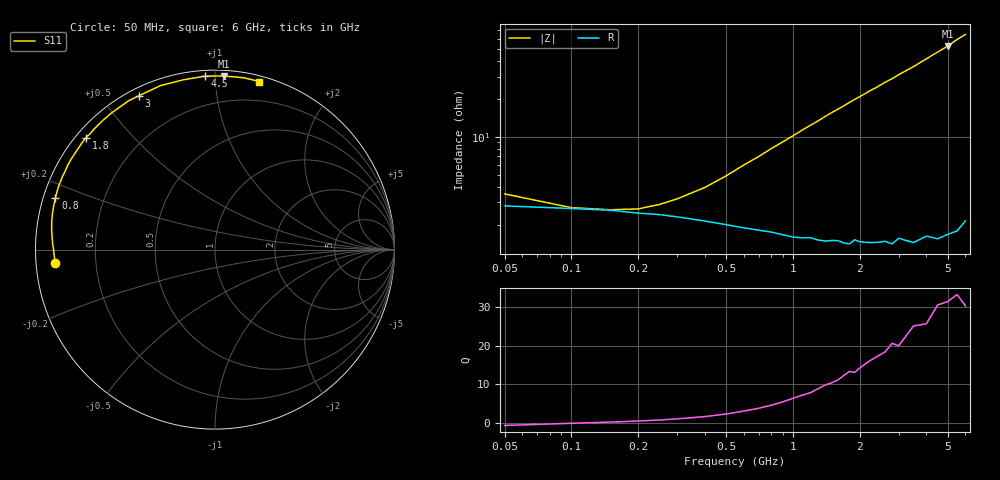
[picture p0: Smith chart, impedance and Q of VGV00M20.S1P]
! Infineon Technologies  Discrete & RF Semiconductors
! BB 831
! Si Tuning Diode in SOD323
! VR =
! S-Parameters:  July  1999
# GHz  S  MA  R  50
!  f  S11
! GHz  MAG  ANG
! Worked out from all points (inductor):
!   34 points, 50 MHz to 6 GHz, reference 50 ohm
!   read as one part to ground: L = 1.59 nH near 700 MHz
!   highest Q = 31.4 at 5 GHz (marker M1), where L = 1.67 nH
!   S11 on the Smith chart (normalised r, x): 50 MHz: 0.06, -0.04; 800 MHz: 0.03, +0.16; 1.8 GHz: 0.03, +0.37; 3 GHz: 0.03, +0.62; 4.5 GHz: 0.03, +0.94; 6 GHz: 0.04, +1.30
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0.05  0.8935 -175.2
0.1  0.8981 -178.9
0.15  0.9011 179.2
0.3  0.9121 174.9
0.5  0.9238 169.8
0.6  0.9282 167.1
0.7  0.9315 164.7
0.8  0.9343 162.1
1  0.9405 157.3
1.1  0.942 154.8
1.3  0.9453 150.2
1.4  0.9468 147.8
1.6  0.9477 143.4
1.7  0.9504 141.3
1.8  0.9518 139.0
1.9  0.9489 136.9
2  0.9513 135.0
2.2  0.9535 130.8
2.4  0.9547 127.2
2.6  0.9554 123.3
2.8  0.9587 120.0
3  0.9561 116.3
3.5  0.9629 108.4
4  0.9624 100.5
4.5  0.9678 93.4
5  0.9687 87.1
5.5  0.9708 80.4
6  0.9686 75.2
